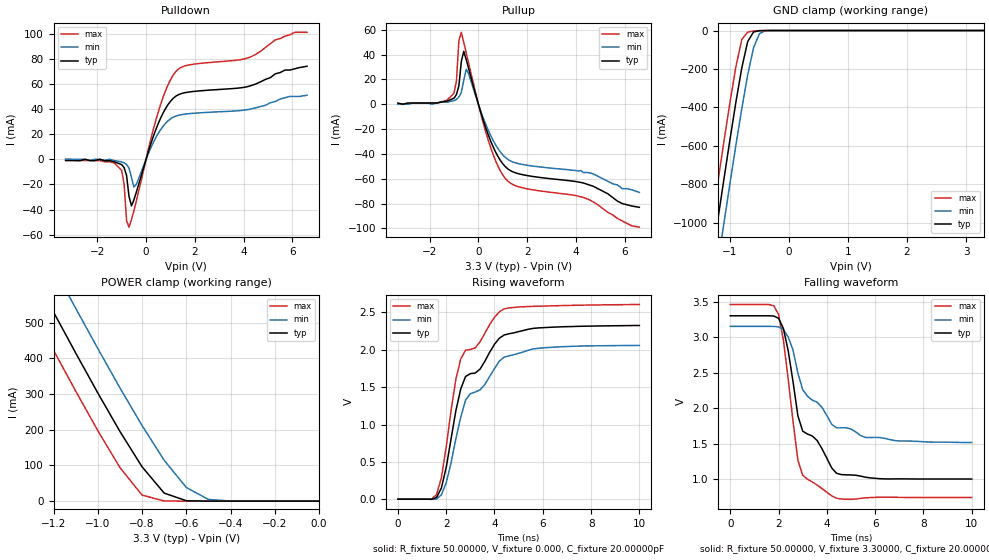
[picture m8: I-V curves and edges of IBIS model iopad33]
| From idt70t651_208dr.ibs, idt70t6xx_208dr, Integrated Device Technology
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|   Model iopad33
[Model]   iopad33
Model_type   I/O
Polarity   Non-Inverting
Enable   Active-Low
Vinl =  0.80000V
Vinh =  2.00000V
Vmeas =  1.50000V
C_comp   4.50000pF   4.50000pF   4.50000pF
[Temperature Range]   25.00000   100.00000   -40.00000
[Voltage Range]   3.30000V   3.10000V   3.50000V
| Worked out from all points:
|   slope of the pulldown table from 0 to 0.495 V, typ, clamps not added: 17.5 ohm
|   slope of the pullup table from 0 to 0.495 V, typ, clamps not added: 16.9 ohm
|   GND clamp passes 1 mA (typ) near -0.50 V on its own axis
|   POWER clamp passes 1 mA (typ) near -0.59 V on its own axis
|   rising waveform, R_fixture 50.00000, V_fixture 0.000, C_fixture 20.00000pF: 20-80 % time 1.6ns typ, 1.66ns min, 1.44ns max; typ from 0 V to 2.33 V
|   falling waveform, R_fixture 50.00000, V_fixture 3.30000, C_fixture 20.00000pF: 20-80 % time 1.36ns typ, 1.49ns min, 578ps max; typ from 3.3 V to 1 V
[Pulldown]
| voltage   I(typ)   I(min)   I(max)
-3.3V     -1mA       0A         0A
-1.5V     -1mA       0A         -2mA
-1V       -4.2mA     -2.1mA     -8.8mA
-900mV    -6.6mA     -2.8mA     -19.8mA
-800mV    -12.8mA    -4.1mA     -48.76mA
-700mV    -29.43mA   -7mA       -53.96mA
-600mV    -37.03mA   -14.17mA   -48.13mA
-500mV    -32.29mA   -22.11mA   -40.89mA
500mV     28.49mA    20.63mA    37.7mA
1.2V      49.93mA    34.24mA    69.32mA
4.1V      57.54mA    39.4mA     80.21mA
6.6V      74mA       51mA       101mA
[Pullup]
| voltage   I(typ)   I(min)   I(max)
-3.3V     1mA        0A         0A
-1.7V     1mA        1mA        1mA
-1V       4.9mA      2.9mA      8.9mA
-900mV    7.8mA      3.9mA      18.89mA
-800mV    14.94mA    5.7mA      51.34mA
-700mV    34.57mA    9.6mA      57.95mA
-600mV    42.62mA    19.25mA    49.81mA
-500mV    36.06mA    28.2mA     41.39mA
400mV     -24.39mA   -20.73mA   -28.72mA
1.1V      -50.2mA    -42.72mA   -59.63mA
4.3V      -63.4mA    -55mA      -75.04mA
6.6V      -83mA      -71mA      -99mA
[GND_clamp]
| voltage   I(typ)   I(min)   I(max)
-3.3V     -5.469A    -5.686A    -5.287A
-1.4V     -1.389A    -1.618A    -1.194A
-1.3V     -1.179A    -1.409A    -984.5mA
-1.2V     -972.3mA   -1.201A    -776.5mA
-1.1V     -767.3mA   -996.6mA   -571.8mA
-900mV    -372.8mA   -596.6mA   -188.1mA
-800mV    -194.3mA   -406.4mA   -47.16mA
-700mV    -57.22mA   -230.7mA   -8.4mA
-600mV    -7.393mA   -88.33mA   -2.169mA
-500mV    -1.009mA   -16.09mA   -229.2uA
-400mV    -92.71uA   -1.476mA   -9.663uA
3.3V      525.2pA    638.3nA    1.93pA
[POWER_clamp]
| voltage   I(typ)   I(min)   I(max)
-3.3V     3.039A     3.158A     2.94A
-1.4V     762.6mA    887.5mA    656.3mA
-1.3V     645.8mA    771mA      539.1mA
-1.2V     529.9mA    655.3mA    422.9mA
-1.1V     415.5mA    540.8mA    308.7mA
-1V       303.3mA    427.9mA    197.7mA
-900mV    195.4mA    317.6mA    94.31mA
-800mV    96.26mA    211.9mA    16.94mA
-700mV    22.53mA    114.6mA    305uA
-600mV    1.137mA    38.18mA    3.7uA
-500mV    27.9uA     4.729mA    76.79nA
0V        525.2pA    48.85nA    2.005pA
[Ramp]
| variable   typ   min   max
dV/dt_r   1.40040/0.58697n   1.23900/0.67661n   1.57020/0.47445n
dV/dt_f   1.38174/0.37674n   1.05360/0.46010n   1.62528/0.29291n
R_load = 50.00000
[Rising Waveform]
R_fixture = 50.00000
V_fixture = 0.000
C_fixture = 20.00000pF
R_dut = 0.19600
L_dut = 13.10000nH
C_dut = 1.92000pF
| time   V(typ)   V(min)   V(max)
0s        0V         0V         0V
1.6ns     23.28mV    2.576mV    63.71mV
2ns       424.9mV    218.8mV    699.6mV
2.4ns     1.185V     807.5mV    1.607V
2.6ns     1.474V     1.097V     1.876V
2.8ns     1.643V     1.326V     1.995V
3.4ns     1.741V     1.464V     2.106V
4.2ns     2.155V     1.848V     2.509V
5.8ns     2.293V     2.02V      2.584V
10ns      2.326V     2.059V     2.607V
[Falling Waveform]
R_fixture = 50.00000
V_fixture = 3.30000
C_fixture = 20.00000pF
R_dut = 0.19600
L_dut = 13.10000nH
C_dut = 1.92000pF
| time   V(typ)   V(min)   V(max)
0s        3.3V       3.151V     3.459V
1.6ns     3.3V       3.151V     3.459V
2ns       3.265V     3.143V     3.32V
2.2ns     3.122V     3.107V     2.959V
2.4ns     2.808V     3.002V     2.408V
2.8ns     1.894V     2.494V     1.27V
3.2ns     1.635V     2.167V     998.5mV
4.6ns     1.064V     1.723V     721mV
5.6ns     1.027V     1.587V     737mV
10ns      1.002V     1.516V     741.8mV
